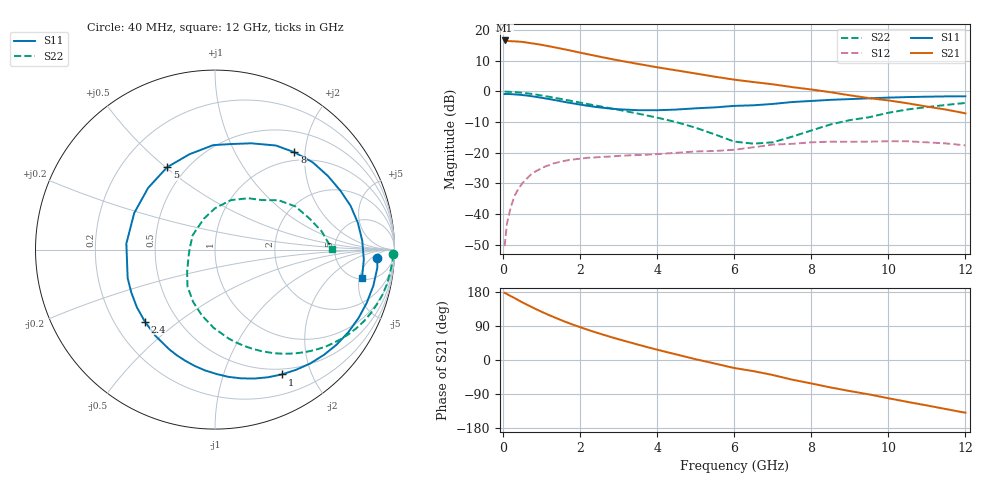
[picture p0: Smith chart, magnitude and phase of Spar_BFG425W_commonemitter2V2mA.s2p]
! Filename: 22bfg425.001
! BFG425W Field C1
! V1=8.063E-001V,V2=2.000E+000V, I1=2.573E-005A, I2=2.000E-003A
# GHz  S  MA  R 50
!  S11  S21  S12  S22
!Freq(GHz)  Mag  Ang  Mag  Ang  Mag  Ang  Mag  Ang
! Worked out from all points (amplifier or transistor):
!   44 points, 40 MHz to 12 GHz, reference 50 ohm
!   highest |S21| = 16.6 dB at 40 MHz (marker M1)
!   |S21| within 3 dB of that: start of sweep to 1.638 GHz
!   unconditionally stable (mu >= 1): 3.122 GHz to end of sweep
!   at 700 MHz: K = 0.18, MSG = 21.6 dB, |S12| = -27.3 dB
!   at 2.4 GHz: K = 0.72, MSG = 16.6 dB, |S12| = -21.5 dB
!   at 12 GHz: K = 1.78, MAG = 0.1 dB, |S12| = -17.6 dB
!   lowest NFmin = 0.80 dB at 900 GHz
!   S11 on the Smith chart (normalised r, x): 40 MHz: 16, -8; 1 GHz: 0.43, -1.58; 2.4 GHz: 0.33, -0.38; 5 GHz: 0.40, +0.51; 8 GHz: 0.84, +1.79; 12 GHz: 5.33, -5.47
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0.04  0.906 -2.9  6.789 177.3  0.003 76.6  0.992 -1.5
0.1  0.91 -6.4  6.658 174.2  0.007 85.9  0.991 -3.8
0.2  0.905 -12.8  6.61 168.5  0.013 81.1  0.984 -7.7
0.3  0.896 -19.3  6.563 163.5  0.02 77.0  0.977 -11.4
0.5  0.874 -31.8  6.429 152.1  0.032 68.8  0.952 -18.8
0.8  0.827 -50.1  6.027 137.0  0.048 57.2  0.901 -29.2
1  0.789 -61.9  5.755 127.3  0.056 50.3  0.86 -35.5
1.2  0.751 -73.1  5.447 118.2  0.063 44.0  0.819 -41.4
1.5  0.693 -89.3  5.002 105.6  0.072 35.6  0.755 -49.3
1.8  0.641 -105.0  4.574 93.8  0.077 28.5  0.696 -56.5
2.2  0.584 -124.6  4.044 79.7  0.083 20.7  0.624 -65.2
2.4  0.56 -134.2  3.812 73.1  0.084 17.4  0.591 -69.3
3  0.512 -161.9  3.21 54.7  0.089 9.5  0.502 -81.2
3.5  0.495 176.1  2.813 40.6  0.092 4.5  0.436 -91.0
4.5  0.507 137.3  2.206 14.6  0.1 -4.1  0.316 -112.7
5  0.531 120.1  1.964 2.0  0.105 -9.6  0.256 -126.8
6  0.582 91.1  1.558 -21.2  0.112 -19.9  0.152 -165.6
6.5  0.595 81.3  1.424 -29.4  0.123 -18.0  0.141 177.5
8  0.7 50.7  1.077 -61.9  0.148 -41.5  0.231 89.7
8.5  0.73 41.8  0.973 -72.4  0.152 -50.4  0.29 72.1
10.5  0.81 10.6  0.642 -110.6  0.154 -84.2  0.509 28.1
12  0.834 -10.8  0.44 -139.1  0.132 -114.9  0.65 0.5
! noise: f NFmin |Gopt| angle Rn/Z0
900  0.8  0.48  17.8  0.27
2000  1.2  0.43  57.2  0.25
